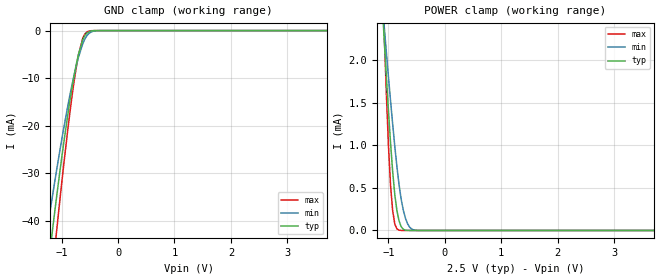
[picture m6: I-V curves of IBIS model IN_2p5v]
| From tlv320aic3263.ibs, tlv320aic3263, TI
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|   IN_2p5v
[Model]   IN_2p5v
Model_type   Input
Vinl = 0.75
Vinh = 1.75
|   typ   min   max
C_comp   1.095pF   1.082pF   1.133pF
[Voltage Range]   2.5   2.25   2.75
[Temperature Range]   27   125   -40
[Power Clamp Reference]   2.5   2.25   2.75
[GND Clamp Reference]   -0   -0   -0
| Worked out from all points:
|   GND clamp passes 1 mA (typ) near -0.58 V on its own axis
|   POWER clamp passes 1 mA (typ) near -0.96 V on its own axis
[GND Clamp]
|   Voltage   I(typ)   I(min)   I(max)
-2.5V     -394.5mA   -329.6mA   -444mA
-1.262V   -52.04mA   -42.59mA   -62.89mA
-1.15V    -40.89mA   -33.94mA   -49.39mA
-1.113V   -37.29mA   -31.15mA   -45.01mA
-1.075V   -33.77mA   -28.41mA   -40.7mA
-887.5mV  -17.49mA   -15.72mA   -20.59mA
-737.5mV  -7.01mA    -7.302mA   -7.558mA
-700mV    -4.978mA   -5.577mA   -5.08mA
-625mV    -1.96mA    -2.786mA   -1.625mA
-550mV    -490.7uA   -1.046mA   -282.7uA
-325mV    -818.2nA   -10.58uA   -58.62nA
4.963V    0A         0A         0A
[POWER Clamp]
|   Voltage   I(typ)   I(min)   I(max)
-2.5V     20.66mA    14.8mA     34.71mA
-1.113V   2.682mA    2.698mA    3.063mA
-1.075V   2.242mA    2.395mA    2.317mA
-1V       1.406mA    1.805mA    1mA
-962.5mV  1.026mA    1.521mA    525.7uA
-925mV    689.7uA    1.247mA    231.4uA
-887.5mV  421uA      988.2uA    76.85uA
-812.5mV  113.7uA    540.4uA    3.334uA
-700mV    3.933uA    146.5uA    8.601nA
-625mV    262.6nA    39.28uA    0A
-512.5mV  4.125nA    2.432uA    0A
4.963V    0A         0A         0A
